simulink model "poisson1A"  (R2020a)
settings: Solver=FixedStepDiscrete  StartTime=0.0  StopTime=100  FixedStep=0.01  MaxStep=0.01  RelTol=1e-3  EnableMultiTasking=on

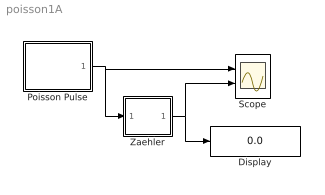
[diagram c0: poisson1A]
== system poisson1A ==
  Display : Display
  Poisson Pulse : Subsystem  mask{lambda=0.8}
  Scope : Scope  NumInputPorts=2
  Zaehler : Subsystem  mask(Vorwaertszaehler){z0=0}
      mask prompts: z0 "Anfangswert"
      mask help: Einfacher Vorwaertszaehler, getriggert durch Signalabfall
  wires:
  Zaehler/1(Out) -> Scope/2, Display/1
  Poisson Pulse/1(Out) -> Scope/1, Zaehler/1(In)

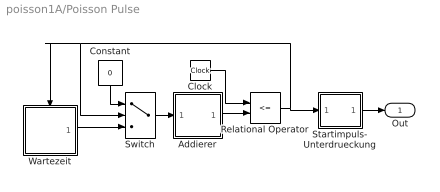
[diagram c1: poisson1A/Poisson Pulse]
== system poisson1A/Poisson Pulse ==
  Addierer : Subsystem
  Clock : Clock
  Constant : Constant  Value=0
  Relational Operator : RelationalOperator  Operator=<=  OutDataTypeStr=boolean
  Startimpuls- Unterdrueckung : Subsystem
  Switch : Switch  Threshold=1
  Wartezeit : Subsystem
  Out : Outport
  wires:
  Clock/1 -> Relational Operator/1
  Relational Operator/1 -> Startimpuls- Unterdrueckung/1(In), Wartezeit/Trigger, Switch/2
  Addierer/1(Summe) -> Relational Operator/2
  Switch/1 -> Addierer/1(In)
  Wartezeit/1(dt) -> Switch/3
  Constant/1 -> Switch/1
  Startimpuls- Unterdrueckung/1(Out) -> Out/1

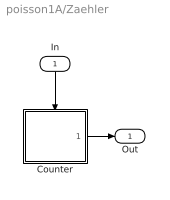
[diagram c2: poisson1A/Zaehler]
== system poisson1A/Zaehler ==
  In : Inport
  Counter : Subsystem
  Out : Outport
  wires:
  In/1 -> Counter/Trigger
  Counter/1(Out) -> Out/1

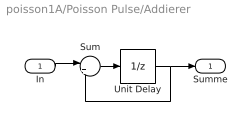
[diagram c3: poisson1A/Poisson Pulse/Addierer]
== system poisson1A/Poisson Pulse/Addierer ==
  In : Inport
  Sum : Sum  Inputs=|++
  Unit Delay : UnitDelay  SampleTime=-1  HasFrameUpgradeWarning=on
  Summe : Outport
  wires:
  Sum/1 -> Unit Delay/1
  Unit Delay/1 -> Summe/1, Sum/2
  In/1 -> Sum/1

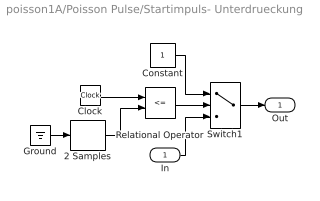
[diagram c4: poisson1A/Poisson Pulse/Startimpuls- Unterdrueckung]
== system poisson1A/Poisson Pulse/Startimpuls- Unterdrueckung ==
  In : Inport
  2 Samples : SampleTimeMath  TsampMathOp=Ts Only  weightValue=2
  Clock : Clock
  Constant : Constant
  Ground : Ground
  Relational Operator : RelationalOperator  Operator=<=  OutDataTypeStr=boolean
  Switch1 : Switch  Threshold=1
  Out : Outport
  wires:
  In/1 -> Switch1/3
  Constant/1 -> Switch1/1
  Relational Operator/1 -> Switch1/2
  Switch1/1 -> Out/1
  Clock/1 -> Relational Operator/1
  2 Samples/1 -> Relational Operator/2
  Ground/1 -> 2 Samples/1

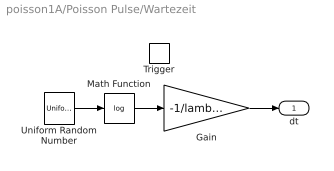
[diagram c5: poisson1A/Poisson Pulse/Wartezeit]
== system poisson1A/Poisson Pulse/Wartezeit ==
  Trigger : TriggerPort  TriggerType=falling  VariantControl=Variant
  Gain : Gain  Gain=-1/lambda
  Math Function : Math  Operator=log  SignedPower=on
  Uniform Random Number : UniformRandomNumber  Minimum=0
  dt : Outport
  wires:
  Uniform Random Number/1 -> Math Function/1
  Math Function/1 -> Gain/1
  Gain/1 -> dt/1

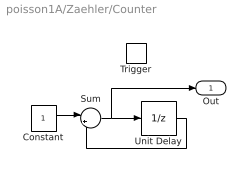
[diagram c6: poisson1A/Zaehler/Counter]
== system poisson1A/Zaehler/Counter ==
  Trigger : TriggerPort  TriggerType=falling  VariantControl=Variant
  Constant : Constant
  Sum : Sum  Inputs=|++
  Unit Delay : UnitDelay  InitialCondition=z0  SampleTime=-1  HasFrameUpgradeWarning=on
  Out : Outport  InitialOutput=z0
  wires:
  Unit Delay/1 -> Sum/2
  Sum/1 -> Out/1, Unit Delay/1
  Constant/1 -> Sum/1
